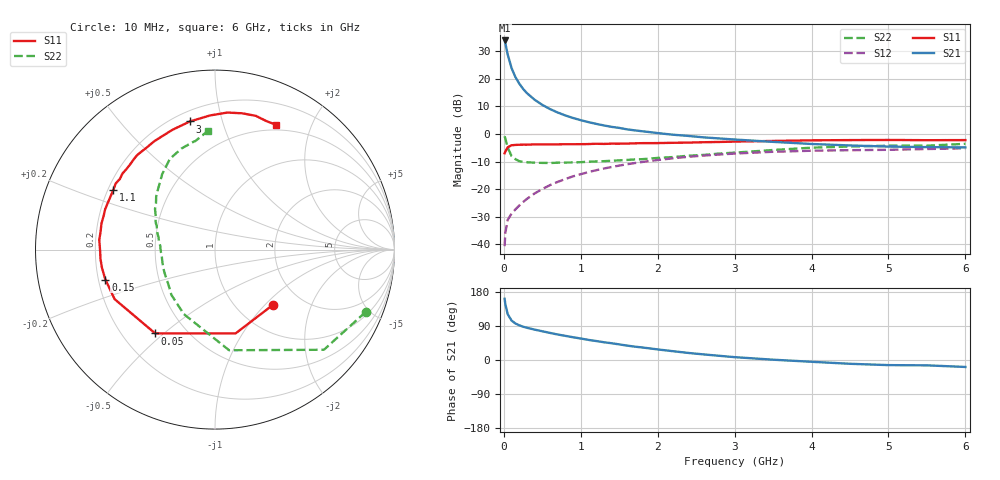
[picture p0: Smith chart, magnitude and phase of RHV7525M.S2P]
! SIEMENS Small Signal Semiconductors
! BFR106
! Si NPN RF Bipolar Junction Transistor in SOT23
! VCE = 0.75 V  IC = 25 mA
! Common Emitter S-Parameters:  August  1996
# GHz  S  MA  R  50
!  f  S11  S21  S12  S22
! GHz  MAG  ANG  MAG  ANG  MAG  ANG  MAG  ANG
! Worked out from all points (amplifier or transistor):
!   36 points, 10 MHz to 6 GHz, reference 50 ohm
!   highest |S21| = 33.9 dB at 10 MHz (marker M1)
!   |S21| within 3 dB of that: start of sweep to 34.37 MHz
!   unconditionally stable (mu >= 1): 284.4 MHz to end of sweep
!   at 250 MHz: K = 0.97, MSG = 20.5 dB, |S12| = -24.7 dB
!   at 1.4 GHz: K = 1.09, MAG = 5.4 dB, |S12| = -12.0 dB
!   at 6 GHz: K = 1.03, MAG = -0.8 dB, |S12| = -5.2 dB
!   S11 on the Smith chart (normalised r, x): 10 MHz: 1.46, -1.11; 50 MHz: 0.34, -0.47; 150 MHz: 0.23, -0.13; 1.1 GHz: 0.22, +0.26; 3 GHz: 0.26, +0.79; 6 GHz: 0.44, +1.52
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0.01  0.4465 -43.3  49.31 161.5  0.0093 76.8  0.9086 -22.5
0.02  0.4809 -76.2  43.47 147.0  0.0165 64.9  0.8244 -42.6
0.05  0.5736 -125.5  27.5 120.9  0.0278 48.9  0.5663 -82.0
0.1  0.6236 -153.7  15.68 104.2  0.0362 47.5  0.399 -115.8
0.15  0.6332 -164.7  10.74 96.4  0.043 50.3  0.3504 -133.9
0.2  0.6379 -170.9  8.188 91.6  0.0505 54.5  0.3219 -144.4
0.25  0.6403 -175.5  6.551 87.9  0.0585 57.5  0.3117 -152.7
0.3  0.6397 -178.8  5.487 85.1  0.0668 59.5  0.3076 -157.6
0.4  0.6471 175.2  4.167 80.2  0.0838 62.1  0.302 -165.5
0.5  0.6453 171.1  3.358 75.8  0.1007 63.2  0.2993 -170.9
0.6  0.649 167.0  2.822 71.5  0.1184 63.2  0.2981 -174.4
0.7  0.6484 163.0  2.447 67.3  0.1357 62.9  0.3018 -177.5
0.9  0.6515 156.6  1.945 60.0  0.1709 60.9  0.3048 176.5
1.1  0.6565 149.7  1.638 53.1  0.204 58.3  0.3143 172.4
1.3  0.6601 143.4  1.427 46.9  0.2367 55.0  0.3216 167.8
1.6  0.6697 135.1  1.213 38.1  0.2826 50.2  0.339 162.1
2.2  0.692 119.4  0.969 23.2  0.3629 39.8  0.3818 150.0
3  0.7274 101.1  0.793 7.5  0.4418 26.1  0.4589 134.1
3.5  0.7477 92.2  0.719 0.8  0.4758 18.4  0.5124 125.1
4.5  0.7744 78.7  0.619 -10.0  0.5084 4.6  0.5935 108.3
5.5  0.7709 68.0  0.579 -14.1  0.5337 -3.6  0.6143 100.3
6  0.7746 63.8  0.571 -18.4  0.5502 -9.9  0.6627 93.4
